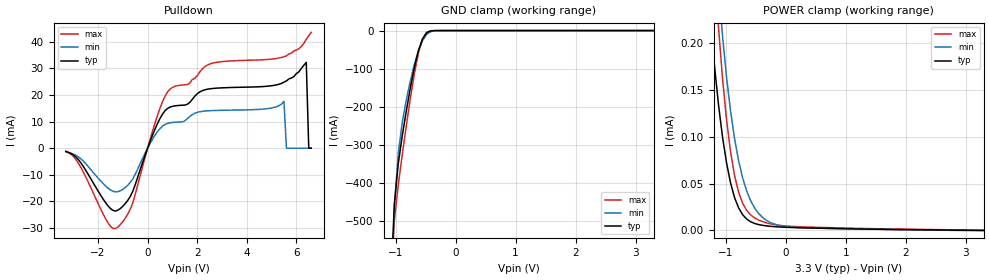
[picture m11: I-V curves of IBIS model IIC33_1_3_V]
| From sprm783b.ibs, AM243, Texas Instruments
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|   Model IIC33_1_3_V
[Model]  IIC33_1_3_V
Model_type I/O_open_drain
Polarity   Non-Inverting
Enable   Active-High
Vinl =  0.990V
Vinh =  2.310V
Vmeas =  1.650V
Cref =  50.000pF
Rref =  1.000M
Vref =  0.0V
C_comp   6.002pF   5.980pF   6.005pF
[Model Spec]
Vinh   2.310V   2.079V   2.541V
Vinl   0.990V   0.891V   1.089V
Vmeas   1.650V   NA   NA
Vref   0.0V   NA   NA
Cref   50.000pF   NA   NA
Rref   1.000M   NA   NA
[Temperature Range]   25.000   0.125k   -40.000
[Voltage Range]   3.300V   2.970V   3.630V
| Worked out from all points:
|   slope of the pulldown table from 0 to 0.495 V, typ, clamps not added: 44.6 ohm
|   GND clamp passes 1 mA (typ) near -0.42 V on its own axis
|   POWER clamp passes 1 mA (typ) near -1.87 V on its own axis
[Pulldown]
|Voltage   I(typ)   I(min)   I(max)
-3.3V     -1.237mA   -1.329mA   -1.147mA
-2.8V     -4.213mA   -3.218mA   -5.535mA
-1.7V     -20.45mA   -14.19mA   -26.45mA
-1.3V     -23.64mA   -16.44mA   -30.29mA
-600mV    -16.25mA   -11.57mA   -20.58mA
700mV     14.06mA    8.936mA    19.5mA
2.3V      21.95mA    13.97mA    30.62mA
5.5V      24.84mA    17.63mA    34.4mA
5.6V      25.35mA    -3.1nA     34.77mA
6.4V      32.3mA     -800nA     40.98mA
6.5V      -100nA     -1uA       42.39mA
6.6V      -200nA     -5uA       43.59mA
[GND_clamp]
|Voltage   I(typ)   I(min)   I(max)
-3.3V     -44.71A    -41.78A    -47.63A
-1.089V   -701.8mA   -759mA     -699.7mA
-1.022V   -456.1mA   -464.3mA   -499.5mA
-955mV    -347.7mA   -319.9mA   -403.8mA
-888mV    -274.3mA   -239.2mA   -324mA
-821mV    -209.8mA   -180.9mA   -248.7mA
-687mV    -96.09mA   -88.17mA   -112.2mA
-620mV    -52.41mA   -52.78mA   -58.95mA
-553mV    -22.16mA   -26.73mA   -22.67mA
-486mV    -6.181mA   -10.55mA   -4.967mA
-285mV    -10.13uA   -113uA     -1.594uA
3.3V      0A         0A         0A
[POWER_clamp]
|Voltage   I(typ)   I(min)   I(max)
-3.266V   6.374A     1.828A     18.01A
-1.256V   225.2uA    392.2uA    358.5uA
-1.122V   134.5uA    260.2uA    217.3uA
-1.055V   99.94uA    207.9uA    162.7uA
-988mV    72.22uA    163.9uA    118.5uA
-921mV    50.87uA    127.6uA    84.13uA
-854mV    35.18uA    98.07uA    58.72uA
-720mV    16.94uA    56.36uA    29.14uA
-586mV    9.315uA    31.79uA    16.69uA
-318mV    4.878uA    10.61uA    8.054uA
17mV      3.368uA    4.051uA    4.707uA
3.3V      0A         0A         270nA
[Ramp]
| variable   typ   min   max
dV/dt_r   0.651/0.103n   0.418/0.146n   0.881/79.852p
dV/dt_f   0.642/6.986n   0.395/8.869n   0.880/4.626n
R_load = 50.000
|End [Component]
| *************************** End IIC_V_3.3V ***************************
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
